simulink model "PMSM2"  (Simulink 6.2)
settings: Solver=ode23  StartTime=0  StopTime=2  FixedStep=0.000001  RelTol=1e-3
undefined symbols (not defined in the file or in its folder): DiscIntNeverNeededParam, J, Lsx, Lsy, p, Psim, Rs, Ts, Udc
libraries: simulink x3

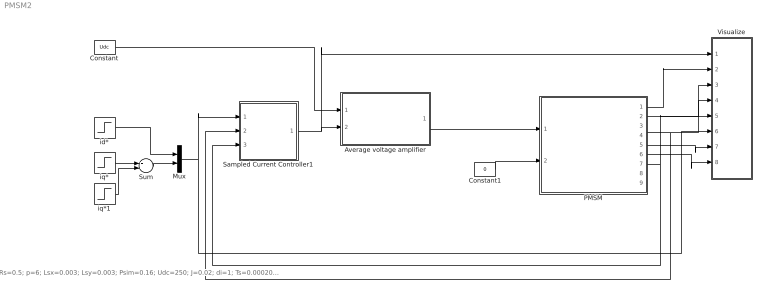
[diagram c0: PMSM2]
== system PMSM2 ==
  note: Rs=0.5; p=6; Lsx=0.003; Lsy=0.003; Psim=0.16; Udc=250; J=0.02; di=1; Ts=0.0002083;
  Average voltage amplifier : Subsystem
  Constant : Constant  Value=Udc
  Constant1 : Constant  Value=0
  Mux : Mux  Inputs=2
  PMSM : Subsystem  mask{Psim=Psim, p=p, Rs=Rs, isy=[0 1], psisy=[0 Lsy], isx=[0 1], psisx=[0 Lsx], J=J}
      mask prompts: p "Number of poles"; Rs "Stator resistance"; isy "y-axis current vector"; psisy "y-axis flux vector"; isx "x-axis current vector"; psisx "x-axis flux vector"; J "Inertia"
  Sampled Current Controller1 : Subsystem  mask{R=Rs, Lx=Lsx, Ly=Lsy, Kp=[(Lsx/Ts+Rs/2) (Lsy/Ts+Rs/2)]', Ti=[(Lsx/Rs+Ts/2) (Lsy/Rs+Ts/2)]', Ts=Ts, Umax=Udc, Umin=-Udc, SlowFast=Fast computer}
      mask prompts: R "Load resistance"; Lx "x-axis load inductance"; Ly "y-axis load inductance"; Kp "Controller gain"; Ti "Integral Time Constant"; Ts "Sampling time [s]"; Umax "Max output signal"; Umin "Min output signal"; SlowFast "Controller type"
  Sum : Sum
  Visualize : Subsystem
  id* : Step  Time=0.0105  After=0  SampleTime=0
  iq* : Step  Time=0.0055  After=10  SampleTime=0
  iq*1 : Step  Time=0.05  After=0  SampleTime=0
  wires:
  Average voltage amplifier/1(vabc) -> PMSM/1(vabc)
  Sampled Current Controller1/1(u*) -> Visualize/1(u*), Average voltage amplifier/2(uabc*)
  Constant/1 -> Average voltage amplifier/1(Udc)
  id*/1 -> Mux/1
  Mux/1 -> Visualize/6(i*dq), Sampled Current Controller1/1(Ref_dq)
  PMSM/7(theta_el) -> Visualize/5(theta), Sampled Current Controller1/3(thetaR)
  Constant1/1 -> PMSM/2(Tl)
  PMSM/1(uabc) -> Visualize/2("u ")
  PMSM/4(is) -> Visualize/4(i), Sampled Current Controller1/2(Act_ab)
  PMSM/2(exy) -> Visualize/3(e)
  PMSM/5(T_mech) -> Visualize/7(Tmech)
  PMSM/6(w_mech) -> Visualize/8(wmech)
  iq*/1 -> Sum/1
  iq*1/1 -> Sum/2
  Sum/1 -> Mux/2

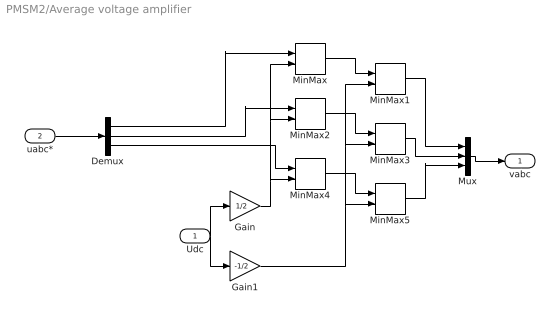
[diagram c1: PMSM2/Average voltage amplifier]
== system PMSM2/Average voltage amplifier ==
  Udc : Inport  Port=1  LatchInput=off
  uabc* : Inport  Port=2  LatchInput=off
  Demux : Demux  Outputs=3
  Gain : Gain  Gain=1/2
  Gain1 : Gain  Gain=-1/2
  MinMax : MinMax  Inputs=2
  MinMax1 : MinMax  Function=max  Inputs=2
  MinMax2 : MinMax  Inputs=2
  MinMax3 : MinMax  Function=max  Inputs=2
  MinMax4 : MinMax  Inputs=2
  MinMax5 : MinMax  Function=max  Inputs=2
  Mux : Mux  Inputs=3
  vabc : Outport  InitialOutput=0
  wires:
  MinMax/1 -> MinMax1/1
  Udc/1 -> Gain/1, Gain1/1
  Gain/1 -> MinMax/2, MinMax2/2, MinMax4/2
  Gain1/1 -> MinMax1/2, MinMax3/2, MinMax5/2
  MinMax2/1 -> MinMax3/1
  MinMax4/1 -> MinMax5/1
  uabc*/1 -> Demux/1
  Demux/1 -> MinMax/1
  Demux/2 -> MinMax2/1
  Demux/3 -> MinMax4/1
  MinMax1/1 -> Mux/1
  MinMax3/1 -> Mux/2
  MinMax5/1 -> Mux/3
  Mux/1 -> vabc/1

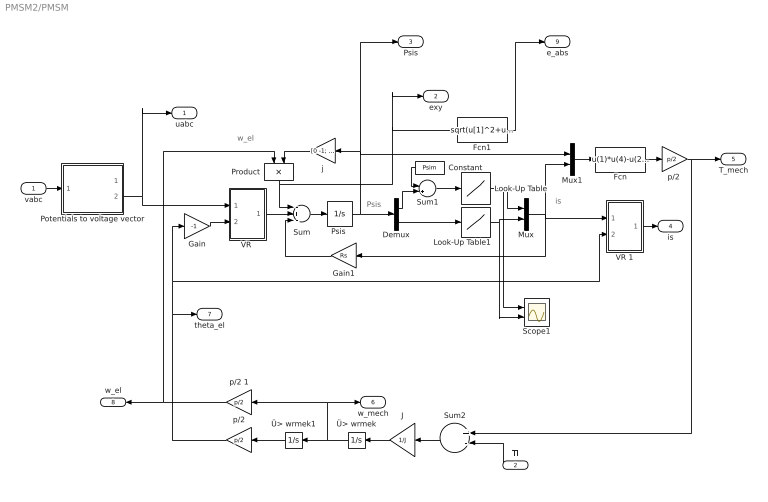
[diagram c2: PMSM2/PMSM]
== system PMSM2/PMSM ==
  note: w_el
  note: Psis
  note: is
  vabc : Inport  Port=1  LatchInput=off
  Tl : Inport  Orientation=left  Port=2  LatchInput=off
  Constant : Constant  Orientation=left  Value=Psim
  Demux : Demux  Outputs=2
  Fcn : Fcn  Expr=u(1)*u(4)-u(2)*u(3)
  Fcn1 : Fcn  Expr=sqrt(u[1]^2+u[2]^2)
  Gain : Gain  Gain=-1
  Gain1 : Gain  Orientation=left  Gain=Rs
  J : Gain  Orientation=left  Gain=1/J
  Look-Up Table : Lookup  InputValues=psisx  OutputValues=isx
  Look-Up Table1 : Lookup  InputValues=psisy  OutputValues=isy
  Mux : Mux  Inputs=2
  Mux1 : Mux  Inputs=2
  Potentials to voltage vector : Subsystem
  Product : Product  Orientation=down
  "Psis " : Integrator  InitialCondition=[Psim 0]'  LimitOutput=on  UpperSaturationLimit=[2*Psim Psim*2]'  LowerSaturationLimit=[Psim/20 0]'
  Scope1 : Scope  NumInputPorts=2
  Sum : Sum  Inputs=-+-
  Sum1 : Sum  Inputs=-+
  Sum2 : Sum  Orientation=left  Inputs=+-
  "VR " : Subsystem
  VR 1 : Subsystem
  j : Gain  Orientation=left  Gain=[0 -1; 1 0]  Multiplication=Matrix(K*u)
  p/2 : Gain  Orientation=left  Gain=p/2  Multiplication=Matrix(K*u)
  "p/2 " : Gain  Gain=p/2  Multiplication=Matrix(K*u)
  p/2 1 : Gain  Orientation=left  Gain=p/2  Multiplication=Matrix(K*u)
  Ü> wrmek : Integrator  Orientation=left
  Ü> wrmek1 : Integrator  Orientation=left
  uabc : Outport
  exy : Outport  Port=2
  Psis : Outport  Port=3
  is : Outport  Port=4
  T_mech : Outport  Port=5
  w_mech : Outport  Port=6
  theta_el : Outport  Port=7
  w_el : Outport  Orientation=left  Port=8
  e_abs : Outport  Port=9
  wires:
  VR 1/1(Out) -> is/1
  Ü> wrmek/1 -> Ü> wrmek1/1, p/2 1/1, w_mech/1
  Fcn1/1 -> e_abs/1
  p/2 1/1 -> w_el/1, Product/1
  Tl/1 -> Sum2/2
  Ü> wrmek1/1 -> p/2/1
  Sum2/1 -> J/1
  J/1 -> Ü> wrmek/1
  vabc/1 -> Potentials to voltage vector/1(In1)
  Potentials to voltage vector/2(uab) -> "VR "/1(vect), uabc/1
  "p/2 "/1 -> Sum2/1, T_mech/1
  Gain/1 -> "VR "/2(angle)
  Sum/1 -> "Psis "/1
  "Psis "/1 -> Demux/1, j/1, Mux1/1, Psis/1
  Demux/1 -> Sum1/2
  Demux/2 -> Look-Up Table1/1
  Look-Up Table/1 -> Scope1/1, Mux/1
  Look-Up Table1/1 -> Scope1/2, Mux/2
  Mux/1 -> Mux1/2, Gain1/1, VR 1/1(vect)
  Mux1/1 -> Fcn/1
  Constant/1 -> Sum1/1
  Sum1/1 -> Look-Up Table/1
  Gain1/1 -> Sum/3
  "VR "/1(Out) -> Sum/2
  Product/1 -> Sum/1, Fcn1/1, exy/1
  Fcn/1 -> "p/2 "/1
  j/1 -> Product/2
  p/2/1 -> theta_el/1, Gain/1, VR 1/2(angle)

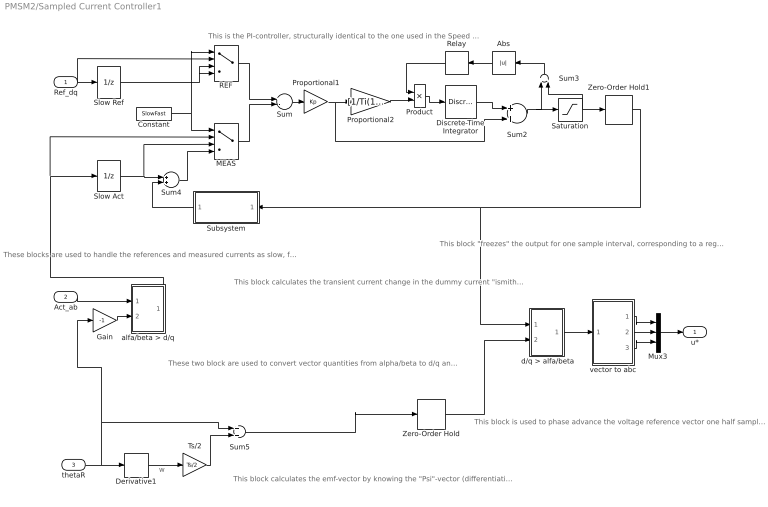
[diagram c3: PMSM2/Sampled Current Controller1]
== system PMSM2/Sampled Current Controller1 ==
  note: These blocks are used to handle the references and measured currents as slow, fast or fast computer with Smith predictor.
  note: This block calculates the transient current change in the dummy current "ismith" The smith predictor calculates the current change that would have been measured if the computer was "fast", i.e. without the delay that a slow computer has. The calculated current change equals the real current change, but informing the controller one sampling interval earlier, thus allowing a high (deadbeat) gain.
  note: This is the PI-controller, structurally identical to the one used in the Speed Controller
  note: This block "freezes" the output for one sample interval, corresponding to a register in a microcontroller where the reference voltages are written once every sampling inteval.
  note: These two block are used to convert vector quantities from alpha/beta to d/q and back again. Note that they are identical, but use the angle with opposite sign.
  note: This block calculates the emf-vector by knowing the "Psi"-vector (differentiation) and calculates the emf- components in the d/q-plane (ideally there is only "eq" whilse "ed"=0). It alse calculates the angle of the "Psi"- vector, used to orient the d/q-plane.
  note: This block is used to phase advance the voltage reference vector one half sample period. It is done to compensate for the fact that the "reality" is turning during the same sample period as the voltage references are being held constant. In the beginning of the sample period, the voltage reference will be 1/2 sample period ahead of reality, and in the end of the sample period it will be 1/2 period behind. In average, it will be in the correct position relative to reality.
  note: w
  Ref_dq : Inport  Port=1  LatchInput=off
  Act_ab : Inport  Port=2  LatchInput=off
  thetaR : Inport  Port=3  LatchInput=off
  " d/q > alfa/beta" : Subsystem
  Abs : Abs  Orientation=left
  Constant : Constant  Value=SlowFast
  Derivative1 : Derivative
  Discrete-Time Integrator : DiscreteIntegrator  SampleTime=Ts  LimitOutput=on  UpperSaturationLimit=Umax  LowerSaturationLimit=Umin  ICPrevOutput=DiscIntNeverNeededParam  ICPrevScaledInput=DiscIntNeverNeededParam
  Gain : Gain  Gain=-1
  MEAS : MultiPortSwitch  Inputs=3
  Mux3 : Mux  Inputs=3
  Product : Product
  Proportional1 : Gain  Gain=Kp
  Proportional2 : Gain  Gain=[1/Ti(1) 1/Ti(2)]
  REF : MultiPortSwitch  Inputs=3
  Relay : Relay  Orientation=left  OnOutputValue=0  OffOutputValue=1
  Saturation : Saturate  UpperLimit=Umax  LowerLimit=Umin
  Slow Act : UnitDelay  SampleTime=Ts
  Slow Ref : UnitDelay  SampleTime=Ts
  Subsystem : Subsystem  Orientation=left
  Sum : Sum  Inputs=+-
  Sum2 : Sum
  Sum3 : Sum  Orientation=up  Inputs=+-
  Sum4 : Sum
  Sum5 : Sum
  Ts/2 : Gain  Gain=Ts/2  Multiplication=Matrix(K*u)
  Zero-Order Hold : ZeroOrderHold  SampleTime=Ts
  Zero-Order Hold1 : ZeroOrderHold  SampleTime=Ts
  alfa/beta > d/q : Subsystem
  vector to abc : Subsystem
  u* : Outport
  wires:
  Discrete-Time Integrator/1 -> Sum2/1
  Proportional1/1 -> Proportional2/1, Sum2/2
  Sum/1 -> Proportional1/1
  Sum2/1 -> Saturation/1, Sum3/1
  Saturation/1 -> Zero-Order Hold1/1, Sum3/2
  Proportional2/1 -> Product/2
  Product/1 -> Discrete-Time Integrator/1
  Relay/1 -> Product/1
  Ref_dq/1 -> REF/2, Slow Ref/1
  Zero-Order Hold1/1 -> Subsystem/1(u), " d/q > alfa/beta"/1(vect)
  Slow Act/1 -> Sum4/1, MEAS/3
  Subsystem/1(di_smith) -> Sum4/2
  Constant/1 -> MEAS/1, REF/1
  Slow Ref/1 -> REF/3, REF/4
  REF/1 -> Sum/1
  Sum4/1 -> MEAS/4
  MEAS/1 -> Sum/2
  Sum3/1 -> Abs/1
  Abs/1 -> Relay/1
  Gain/1 -> alfa/beta > d/q/2(angle)
  Act_ab/1 -> alfa/beta > d/q/1(vect)
  Sum5/1 -> Zero-Order Hold/1
  Zero-Order Hold/1 -> " d/q > alfa/beta"/2(angle)
  " d/q > alfa/beta"/1(Out) -> vector to abc/1(vect)
  vector to abc/1(a) -> Mux3/1
  vector to abc/2(b) -> Mux3/2
  vector to abc/3(c) -> Mux3/3
  alfa/beta > d/q/1(Out) -> Slow Act/1, MEAS/2
  Mux3/1 -> u*/1
  thetaR/1 -> Derivative1/1, Gain/1, Sum5/1
  Derivative1/1 -> Ts/2/1
  Ts/2/1 -> Sum5/2

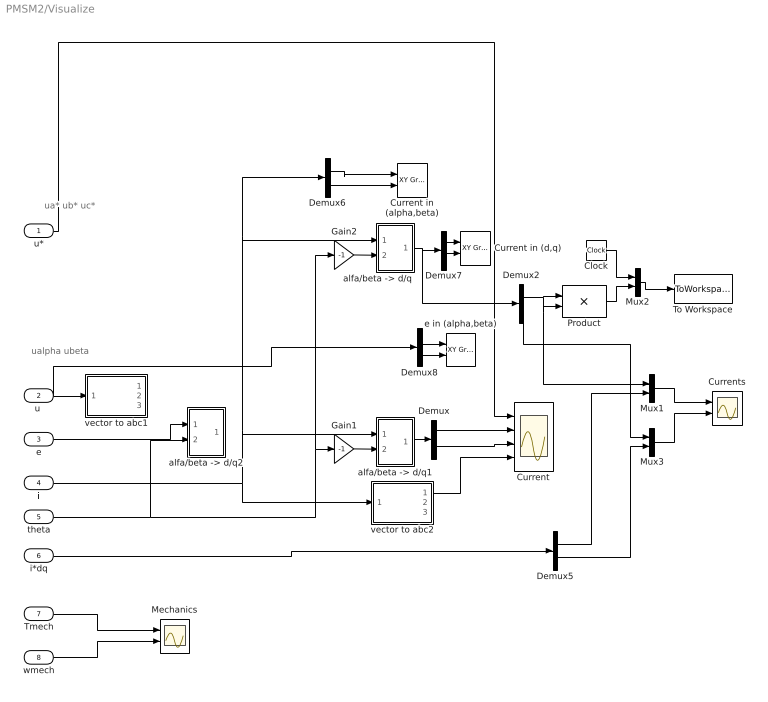
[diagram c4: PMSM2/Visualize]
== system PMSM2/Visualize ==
  note: ua* ub* uc*
  note: ualpha ubeta
  u* : Inport  Port=1  LatchInput=off
  "u " : Inport  Port=2  LatchInput=off
  e : Inport  Port=3  LatchInput=off
  i : Inport  Port=4  LatchInput=off
  theta : Inport  Port=5  LatchInput=off
  i*dq : Inport  Port=6  LatchInput=off
  Tmech : Inport  Port=7  LatchInput=off
  wmech : Inport  Port=8  LatchInput=off
  Clock : Clock
  Current : Scope  NumInputPorts=4
  Current in (alpha,beta) : simulink/Sinks/XY Graph  xmin=-20  xmax=20  ymin=-20  ymax=20  st=-1
  Current in (d,q) : simulink/Sinks/XY Graph  xmin=-20  xmax=20  ymin=-20  ymax=20  st=-1
  Currents : Scope  NumInputPorts=2
  Demux{,2,5..8} (6 alike) : Demux  Outputs=2
  Gain1 : Gain  Gain=-1
  Gain2 : Gain  Gain=-1
  Mechanics : Scope  NumInputPorts=2
  Mux1 : Mux  Inputs=2
  Mux2 : Mux  Inputs=2
  Mux3 : Mux  Inputs=2
  Product : Product
  To Workspace : ToWorkspace  VariableName=f1  SampleTime=-1  SaveFormat=Array
  "alfa/beta -> d/q" : Subsystem
  "alfa/beta -> d/q1" : Subsystem
  "alfa/beta -> d/q2" : Subsystem
  e in (alpha,beta) : simulink/Sinks/XY Graph  xmin=-300  xmax=300  ymin=-300  ymax=300  st=-1
  vector to abc1 : Subsystem
  vector to abc2 : Subsystem
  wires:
  Gain2/1 -> "alfa/beta -> d/q"/2(angle)
  Gain1/1 -> "alfa/beta -> d/q1"/2(angle)
  "alfa/beta -> d/q1"/1(Out) -> Demux/1
  Demux/1 -> Current/2
  Demux/2 -> Current/3
  vector to abc2/1(a) -> Current/4
  "alfa/beta -> d/q"/1(Out) -> Demux2/1, Demux7/1
  u*/1 -> Current/1
  "u "/1 -> vector to abc1/1(vect), Demux8/1
  i/1 -> "alfa/beta -> d/q"/1(vect), Demux6/1, "alfa/beta -> d/q1"/1(vect), vector to abc2/1(vect)
  theta/1 -> Gain1/1, Gain2/1, "alfa/beta -> d/q2"/2(angle)
  Clock/1 -> Mux2/1
  Product/1 -> Mux2/2
  Mux2/1 -> To Workspace/1
  Demux2/1 -> Product/1, Product/2, Mux1/1
  i*dq/1 -> Demux5/1
  Demux5/1 -> Mux1/2
  Demux2/2 -> Mux3/1
  Demux5/2 -> Mux3/2
  Mux3/1 -> Currents/2
  Mux1/1 -> Currents/1
  e/1 -> "alfa/beta -> d/q2"/1(vect)
  "alfa/beta -> d/q2"/1(Out) -> ?
  Tmech/1 -> Mechanics/1
  wmech/1 -> Mechanics/2
  Demux6/1 -> Current in (alpha,beta)/1
  Demux6/2 -> Current in (alpha,beta)/2
  Demux7/1 -> Current in (d,q)/1
  Demux7/2 -> Current in (d,q)/2
  Demux8/1 -> e in (alpha,beta)/1
  Demux8/2 -> e in (alpha,beta)/2

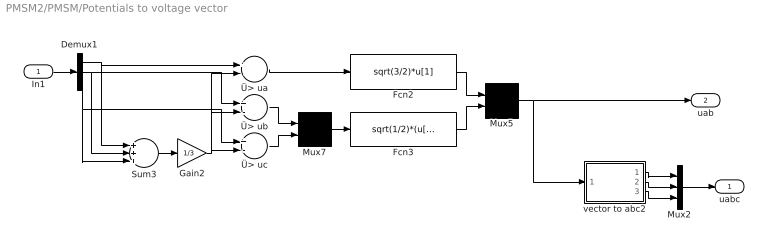
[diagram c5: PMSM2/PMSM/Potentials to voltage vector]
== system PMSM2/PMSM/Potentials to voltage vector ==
  In1 : Inport  Port=1  LatchInput=off
  Demux1 : Demux  Outputs=3
  Fcn2 : Fcn  Expr=sqrt(3/2)*u[1]
  Fcn3 : Fcn  Expr=sqrt(1/2)*(u[1]-u[2])
  Gain2 : Gain  Gain=1/3
  Mux2 : Mux  Inputs=3
  Mux5 : Mux  Inputs=2
  Mux7 : Mux  Inputs=2
  Sum3 : Sum  Inputs=+++
  vector to abc2 : Subsystem
  Ü> ua : Sum  Inputs=+-
  Ü> ub : Sum  Inputs=+-
  Ü> uc : Sum  Inputs=+-
  uabc : Outport
  uab : Outport  Port=2
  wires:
  Fcn3/1 -> Mux5/2
  Fcn2/1 -> Mux5/1
  Mux7/1 -> Fcn3/1
  Ü> uc/1 -> Mux7/2
  Ü> ub/1 -> Mux7/1
  Ü> ua/1 -> Fcn2/1
  Gain2/1 -> Ü> uc/2, Ü> ub/2, Ü> ua/2
  Demux1/2 -> Ü> ub/1, Sum3/2
  Sum3/1 -> Gain2/1
  Demux1/3 -> Ü> uc/1, Sum3/3
  Demux1/1 -> Ü> ua/1, Sum3/1
  In1/1 -> Demux1/1
  Mux5/1 -> uab/1, vector to abc2/1(vect)
  vector to abc2/1(a) -> Mux2/1
  vector to abc2/2(b) -> Mux2/2
  vector to abc2/3(c) -> Mux2/3
  Mux2/1 -> uabc/1

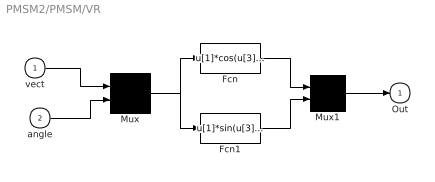
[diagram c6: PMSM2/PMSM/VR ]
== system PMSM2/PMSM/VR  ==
  vect : Inport  Port=1  LatchInput=off
  angle : Inport  Port=2  LatchInput=off
  Fcn : Fcn  Expr=u[1]*cos(u[3])-u[2]*sin(u[3])
  Fcn1 : Fcn  Expr=u[1]*sin(u[3])+u[2]*cos(u[3])
  Mux : Mux  Inputs=2
  Mux1 : Mux  Inputs=2
  Out : Outport  InitialOutput=0
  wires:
  Mux1/1 -> Out/1
  Fcn1/1 -> Mux1/2
  Fcn/1 -> Mux1/1
  Mux/1 -> Fcn1/1, Fcn/1
  angle/1 -> Mux/2
  vect/1 -> Mux/1

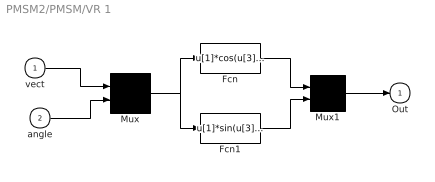
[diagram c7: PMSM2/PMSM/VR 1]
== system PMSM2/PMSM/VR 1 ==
  vect : Inport  Port=1  LatchInput=off
  angle : Inport  Port=2  LatchInput=off
  Fcn : Fcn  Expr=u[1]*cos(u[3])-u[2]*sin(u[3])
  Fcn1 : Fcn  Expr=u[1]*sin(u[3])+u[2]*cos(u[3])
  Mux : Mux  Inputs=2
  Mux1 : Mux  Inputs=2
  Out : Outport  InitialOutput=0
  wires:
  vect/1 -> Mux/1
  angle/1 -> Mux/2
  Mux/1 -> Fcn/1, Fcn1/1
  Fcn/1 -> Mux1/1
  Fcn1/1 -> Mux1/2
  Mux1/1 -> Out/1

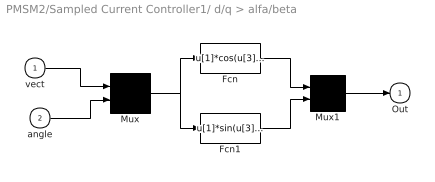
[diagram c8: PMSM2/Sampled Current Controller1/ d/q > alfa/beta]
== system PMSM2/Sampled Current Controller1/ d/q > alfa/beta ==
  vect : Inport  Port=1  LatchInput=off
  angle : Inport  Port=2  LatchInput=off
  Fcn : Fcn  Expr=u[1]*cos(u[3])-u[2]*sin(u[3])
  Fcn1 : Fcn  Expr=u[1]*sin(u[3])+u[2]*cos(u[3])
  Mux : Mux  Inputs=2
  Mux1 : Mux  Inputs=2
  Out : Outport  InitialOutput=0
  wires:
  Mux1/1 -> Out/1
  Fcn1/1 -> Mux1/2
  Fcn/1 -> Mux1/1
  Mux/1 -> Fcn1/1, Fcn/1
  angle/1 -> Mux/2
  vect/1 -> Mux/1

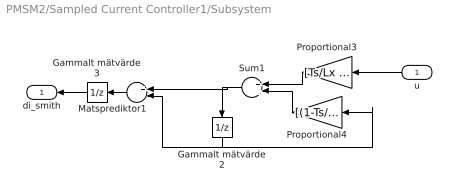
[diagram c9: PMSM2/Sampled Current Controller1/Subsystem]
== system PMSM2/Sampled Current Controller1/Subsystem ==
  u : Inport  Orientation=left  Port=1  LatchInput=off
  Gammalt mätvärde2 : UnitDelay  Orientation=down  SampleTime=Ts
  Gammalt mätvärde3 : UnitDelay  Orientation=left  SampleTime=Ts
  Matsprediktor1 : Sum  Orientation=left  Inputs=+-
  Proportional3 : Gain  Orientation=left  Gain=[Ts/Lx Ts/Ly]
  Proportional4 : Gain  Orientation=left  Gain=[(1-Ts/(Lx/R)) (1-Ts/(Ly/R))]
  Sum1 : Sum  Orientation=left
  di_smith : Outport  Orientation=left
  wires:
  Proportional3/1 -> Sum1/1
  Proportional4/1 -> Sum1/2
  Sum1/1 -> Gammalt mätvärde2/1, Matsprediktor1/1
  u/1 -> Proportional3/1
  Matsprediktor1/1 -> Gammalt mätvärde3/1
  Gammalt mätvärde3/1 -> di_smith/1
  Gammalt mätvärde2/1 -> Proportional4/1, Matsprediktor1/2

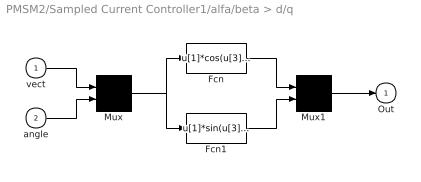
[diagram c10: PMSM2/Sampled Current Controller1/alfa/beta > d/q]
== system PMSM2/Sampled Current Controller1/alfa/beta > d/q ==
  vect : Inport  Port=1  LatchInput=off
  angle : Inport  Port=2  LatchInput=off
  Fcn : Fcn  Expr=u[1]*cos(u[3])-u[2]*sin(u[3])
  Fcn1 : Fcn  Expr=u[1]*sin(u[3])+u[2]*cos(u[3])
  Mux : Mux  Inputs=2
  Mux1 : Mux  Inputs=2
  Out : Outport  InitialOutput=0
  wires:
  vect/1 -> Mux/1
  angle/1 -> Mux/2
  Mux/1 -> Fcn/1, Fcn1/1
  Fcn/1 -> Mux1/1
  Fcn1/1 -> Mux1/2
  Mux1/1 -> Out/1

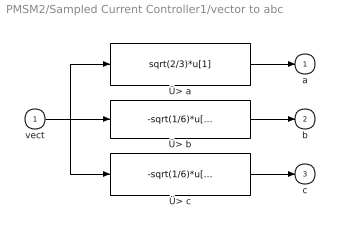
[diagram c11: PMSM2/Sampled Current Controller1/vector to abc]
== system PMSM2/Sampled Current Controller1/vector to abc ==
  vect : Inport  Port=1  LatchInput=off
  Ü> a : Fcn  Expr=sqrt(2/3)*u[1]
  Ü> b : Fcn  Expr=-sqrt(1/6)*u[1]+sqrt(1/2)*u[2]
  Ü> c : Fcn  Expr=-sqrt(1/6)*u[1]-sqrt(1/2)*u[2]
  a : Outport  InitialOutput=0
  b : Outport  Port=2  InitialOutput=0
  c : Outport  Port=3  InitialOutput=0
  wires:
  vect/1 -> Ü> b/1, Ü> a/1, Ü> c/1
  Ü> b/1 -> b/1
  Ü> c/1 -> c/1
  Ü> a/1 -> a/1

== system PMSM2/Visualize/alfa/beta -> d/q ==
  vect : Inport  Port=1  LatchInput=off
  angle : Inport  Port=2  LatchInput=off
  Fcn : Fcn  Expr=u[1]*cos(u[3])-u[2]*sin(u[3])
  Fcn1 : Fcn  Expr=u[1]*sin(u[3])+u[2]*cos(u[3])
  Mux : Mux  Inputs=2
  Mux1 : Mux  Inputs=2
  Out : Outport  InitialOutput=0
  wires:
  vect/1 -> Mux/1
  angle/1 -> Mux/2
  Mux/1 -> Fcn/1, Fcn1/1
  Fcn/1 -> Mux1/1
  Fcn1/1 -> Mux1/2
  Mux1/1 -> Out/1

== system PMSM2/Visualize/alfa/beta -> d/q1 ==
  vect : Inport  Port=1  LatchInput=off
  angle : Inport  Port=2  LatchInput=off
  Fcn : Fcn  Expr=u[1]*cos(u[3])-u[2]*sin(u[3])
  Fcn1 : Fcn  Expr=u[1]*sin(u[3])+u[2]*cos(u[3])
  Mux : Mux  Inputs=2
  Mux1 : Mux  Inputs=2
  Out : Outport  InitialOutput=0
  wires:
  Mux1/1 -> Out/1
  Fcn1/1 -> Mux1/2
  Fcn/1 -> Mux1/1
  Mux/1 -> Fcn1/1, Fcn/1
  angle/1 -> Mux/2
  vect/1 -> Mux/1

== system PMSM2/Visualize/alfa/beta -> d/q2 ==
  vect : Inport  Port=1  LatchInput=off
  angle : Inport  Port=2  LatchInput=off
  Fcn : Fcn  Expr=u[1]*cos(u[3])-u[2]*sin(u[3])
  Fcn1 : Fcn  Expr=u[1]*sin(u[3])+u[2]*cos(u[3])
  Mux : Mux  Inputs=2
  Mux1 : Mux  Inputs=2
  Out : Outport  InitialOutput=0
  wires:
  vect/1 -> Mux/1
  angle/1 -> Mux/2
  Mux/1 -> Fcn/1, Fcn1/1
  Fcn/1 -> Mux1/1
  Fcn1/1 -> Mux1/2
  Mux1/1 -> Out/1

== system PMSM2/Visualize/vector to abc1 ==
  vect : Inport  Port=1  LatchInput=off
  Ü> a : Fcn  Expr=sqrt(2/3)*u[1]
  Ü> b : Fcn  Expr=-sqrt(1/6)*u[1]+sqrt(1/2)*u[2]
  Ü> c : Fcn  Expr=-sqrt(1/6)*u[1]-sqrt(1/2)*u[2]
  a : Outport  InitialOutput=0
  b : Outport  Port=2  InitialOutput=0
  c : Outport  Port=3  InitialOutput=0
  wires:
  Ü> a/1 -> a/1
  Ü> c/1 -> c/1
  Ü> b/1 -> b/1
  vect/1 -> Ü> c/1, Ü> a/1, Ü> b/1

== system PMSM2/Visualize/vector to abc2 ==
  vect : Inport  Port=1  LatchInput=off
  Ü> a : Fcn  Expr=sqrt(2/3)*u[1]
  Ü> b : Fcn  Expr=-sqrt(1/6)*u[1]+sqrt(1/2)*u[2]
  Ü> c : Fcn  Expr=-sqrt(1/6)*u[1]-sqrt(1/2)*u[2]
  a : Outport  InitialOutput=0
  b : Outport  Port=2  InitialOutput=0
  c : Outport  Port=3  InitialOutput=0
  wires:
  vect/1 -> Ü> b/1, Ü> a/1, Ü> c/1
  Ü> b/1 -> b/1
  Ü> c/1 -> c/1
  Ü> a/1 -> a/1

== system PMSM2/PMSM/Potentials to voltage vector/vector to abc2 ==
  vect : Inport  Port=1  LatchInput=off
  Ü> a : Fcn  Expr=sqrt(2/3)*u[1]
  Ü> b : Fcn  Expr=-sqrt(1/6)*u[1]+sqrt(1/2)*u[2]
  Ü> c : Fcn  Expr=-sqrt(1/6)*u[1]-sqrt(1/2)*u[2]
  a : Outport  InitialOutput=0
  b : Outport  Port=2  InitialOutput=0
  c : Outport  Port=3  InitialOutput=0
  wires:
  vect/1 -> Ü> b/1, Ü> a/1, Ü> c/1
  Ü> b/1 -> b/1
  Ü> c/1 -> c/1
  Ü> a/1 -> a/1
